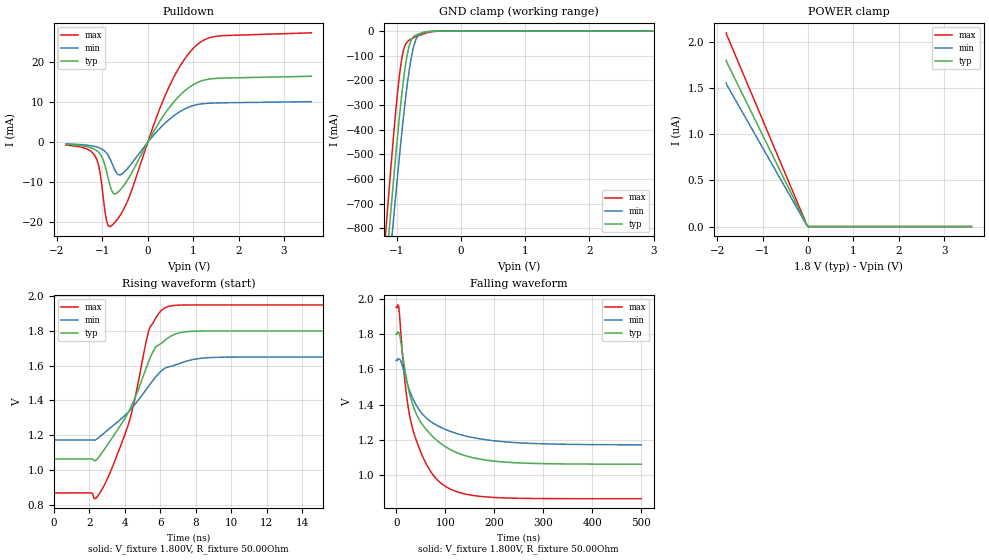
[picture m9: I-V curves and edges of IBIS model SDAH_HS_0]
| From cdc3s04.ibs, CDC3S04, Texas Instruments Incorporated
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|   1.8V Input/Output model
[Model]   SDAH_HS_0
Model_type   I/O_open_sink
Vinl =  540.000mV
Vinh =  1.260V
Vmeas = 0.9
Vref =  1.800V
Cref =  1.000pF   |max
Rref =  1200.000Ohm
|   typ   min   max
C_comp   3.198pF   3.043pF   3.365pF
[Voltage Range]   1.800V   1.650V   1.950V
[Temperature Range]   32.0   85.0   -40.0
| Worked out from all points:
|   slope of the pulldown table from 0 to 0.27 V, typ, clamps not added: 50.8 ohm
|   GND clamp passes 1 mA (typ) near -0.41 V on its own axis
|   falling waveform, V_fixture 1.800V, R_fixture 50.00Ohm: 20-80 % time 63.2ns typ, 74.5ns min, 46.4ns max; typ from 1.8 V to 1.06 V
|   rising waveform, V_fixture 1.800V, R_fixture 50.00Ohm: 20-80 % time 2ns typ, 2.42ns min, 1.63ns max; typ from 1.06 V to 1.8 V
[Pulldown]
|   Voltage   I(typ)   I(min)   I(max)
-1.8V     -552.4uA   -410.7uA   -722.1uA
-1.152V   -1.913mA   -1.119mA   -3.654mA
-1.056V   -2.883mA   -1.479mA   -7.377mA
-913.1mV  -7.084mA   -2.669mA   -19.33mA
-818.6mV  -11.31mA   -4.497mA   -21.01mA
-725.4mV  -12.92mA   -6.918mA   -20.03mA
-560.7mV  -11.29mA   -7.877mA   -17.34mA
404.5mV   7.587mA    5.022mA    12.25mA
716.4mV   11.82mA    7.701mA    19.14mA
1.027V    14.54mA    9.233mA    23.74mA
1.509V    15.94mA    9.801mA    26.45mA
3.599V    16.46mA    10.13mA    27.32mA
[GND Clamp]
|   Voltage   I(typ)   I(min)   I(max)
-1.8V     -3.042A    -3.085A    -3.042A
-1.172V   -976.6mA   -1.122A    -817.1mA
-1.128V   -837.8mA   -989.2mA   -669.4mA
-1.086V   -709.9mA   -866.1mA   -534.7mA
-1.053V   -613.1mA   -772.3mA   -434.3mA
-973.8mV  -387.5mA   -549.4mA   -214.9mA
-915.8mV  -242.4mA   -397.4mA   -103.1mA
-815.9mV  -69.7mA    -176.1mA   -38.76mA
-713.3mV  -17.86mA   -42.34mA   -24.74mA
-640.4mV  -10.49mA   -11.77mA   -16.97mA
-447.3mV  -1.435mA   -776.2uA   -2.631mA
3.599V    0A         0A         0A
[POWER Clamp]
|   Voltage   I(typ)   I(min)   I(max)
-1.8V     1.802uA    1.556uA    2.099uA
-1.799V   1.79uA     1.543uA    2.086uA
-26.1mV   14.13nA    12.14nA    17.55nA
0V        0A         0A         0A
3.599V    0A         0A         0A
[Ramp]
R_load = 50.00Ohm
|   typ   min   max
dV/dt_r   442.506mV/2.005ns   286.699mV/2.415ns   649.678mV/1.632ns
dV/dt_f   442.506mV/63.200ns  286.699mV/74.483ns  649.678mV/46.299ns
[Falling Waveform]
V_fixture = 1.800V
V_fixture_min = 1.650V
V_fixture_max = 1.950V
R_fixture = 50.00Ohm
|   Time   V(typ)   V(min)   V(max)
0s        1.8V       1.65V      1.95V
5.4ns     1.808V     1.658V     1.948V
18.8ns    1.579V     1.556V     1.505V
25.15ns   1.488V     1.498V     1.373V
32.35ns   1.411V     1.445V     1.275V
61.1ns    1.259V     1.325V     1.065V
92.9ns    1.176V     1.268V     951.6mV
131.7ns   1.119V     1.229V     899.8mV
200.6ns   1.08V      1.195V     874.1mV
499.9ns   1.062V     1.172V     867.2mV
[Rising Waveform]
V_fixture = 1.800V
V_fixture_min = 1.650V
V_fixture_max = 1.950V
R_fixture = 50.00Ohm
|   Time   V(typ)   V(min)   V(max)
0s        1.062V     1.172V     867.2mV
2.3ns     1.052V     1.171V     833.7mV
2.55ns    1.076V     1.188V     860mV
3.15ns    1.163V     1.239V     978.5mV
4.2ns     1.331V     1.334V     1.261V
5.4ns     1.638V     1.49V      1.816V
6.15ns    1.737V     1.577V     1.926V
7.25ns    1.793V     1.619V     1.949V
11.65ns   1.8V       1.65V      1.95V
499.9ns   1.8V       1.65V      1.95V
